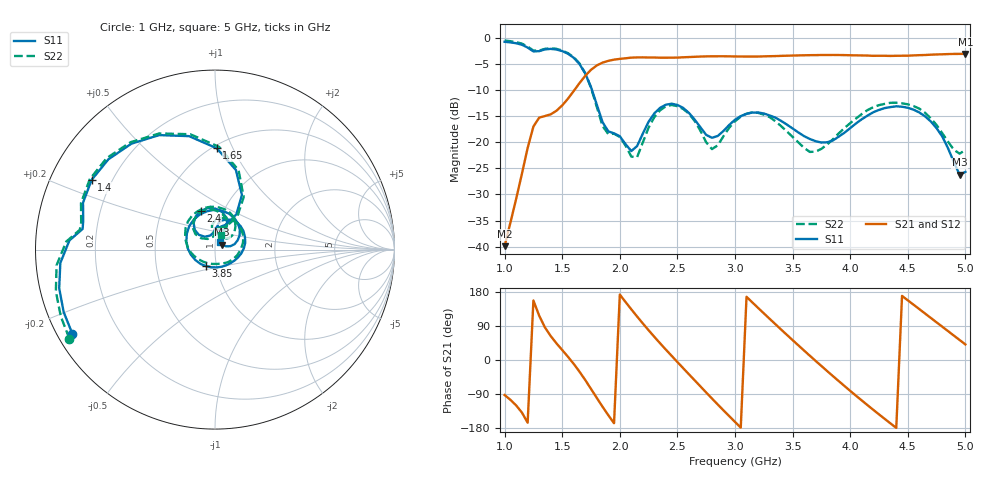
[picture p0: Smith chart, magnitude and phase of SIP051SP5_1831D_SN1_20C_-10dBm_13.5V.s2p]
# GHz  S  dB  R  50
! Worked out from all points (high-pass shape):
!   81 points, 1 GHz to 5 GHz, reference 50 ohm
!   highest |S21| = -3.01 dB at 5 GHz (marker M1); lowest = -39.9 dB at 1 GHz (marker M2)
!   |S21| within 3 dB of the highest: 1.753 GHz to end of sweep
!   lowest |S11| = -26.2 dB at 4.95 GHz (marker M3), VSWR 1.10, Z = 54.1 + j2.95 ohm
!   |S11| at or under -10 dB: 1.759 GHz to end of sweep
!   |S22| runs from -22.8 to -0.4 dB; largest |S21 - S12| = 0.0028
!   S11 on the Smith chart (normalised r, x): 1 GHz: 0.04, -0.27; 1.4 GHz: 0.13, +0.26; 1.65 GHz: 0.52, +0.87; 2.4 GHz: 0.78, +0.36; 3.85 GHz: 0.89, -0.17; 5 GHz: 1.05, +0.09
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1  -0.70 -149.3  -39.92 -92.4  -39.59 -94.1  -0.44 -148.6
1.25  -2.54 171.2  -16.96 157.1  -16.95 157.0  -2.37 171.7
1.4  -2.05 150.5  -14.62 63.3  -14.61 63.1  -1.94 150.7
1.65  -4.96 89.0  -8.62 -30.8  -8.62 -30.7  -4.84 87.7
1.7  -6.77 75.3  -7.22 -52.8  -7.24 -52.9  -6.72 73.5
1.85  -16.11 64.7  -4.69 -123.2  -4.68 -123.3  -16.86 64.3
2  -18.82 90.0  -3.97 172.7  -3.97 172.8  -18.96 88.6
2.2  -18.31 137.5  -3.69 96.4  -3.68 96.4  -20.00 140.7
2.35  -13.37 119.8  -3.75 44.0  -3.74 44.0  -13.85 125.8
2.4  -12.77 110.0  -3.75 27.3  -3.76 27.2  -13.07 114.7
2.55  -13.38 79.9  -3.67 -21.5  -3.68 -21.5  -13.60 81.3
2.75  -18.57 67.1  -3.50 -85.7  -3.49 -85.7  -19.99 65.1
3  -15.65 77.4  -3.51 -163.4  -3.50 -163.4  -15.95 90.1
3.15  -14.28 52.6  -3.53 152.1  -3.53 152.1  -14.24 60.5
3.35  -15.25 12.9  -3.44 94.7  -3.44 94.7  -15.92 13.2
3.7  -19.78 -68.0  -3.25 -2.4  -3.25 -2.4  -21.77 -101.7
3.85  -19.64 -118.0  -3.22 -42.5  -3.23 -42.4  -19.41 -150.3
4.1  -15.57 163.5  -3.31 -106.6  -3.31 -106.7  -14.57 152.8
4.35  -13.23 101.6  -3.41 -167.4  -3.40 -167.3  -12.40 105.2
4.7  -15.99 30.2  -3.17 110.9  -3.17 111.0  -15.40 47.9
4.95  -26.22 33.8  -3.02 52.7  -3.02 52.8  -22.17 57.1
5  -25.67 58.2  -3.01 41.1  -3.02 41.1  -21.47 68.6
